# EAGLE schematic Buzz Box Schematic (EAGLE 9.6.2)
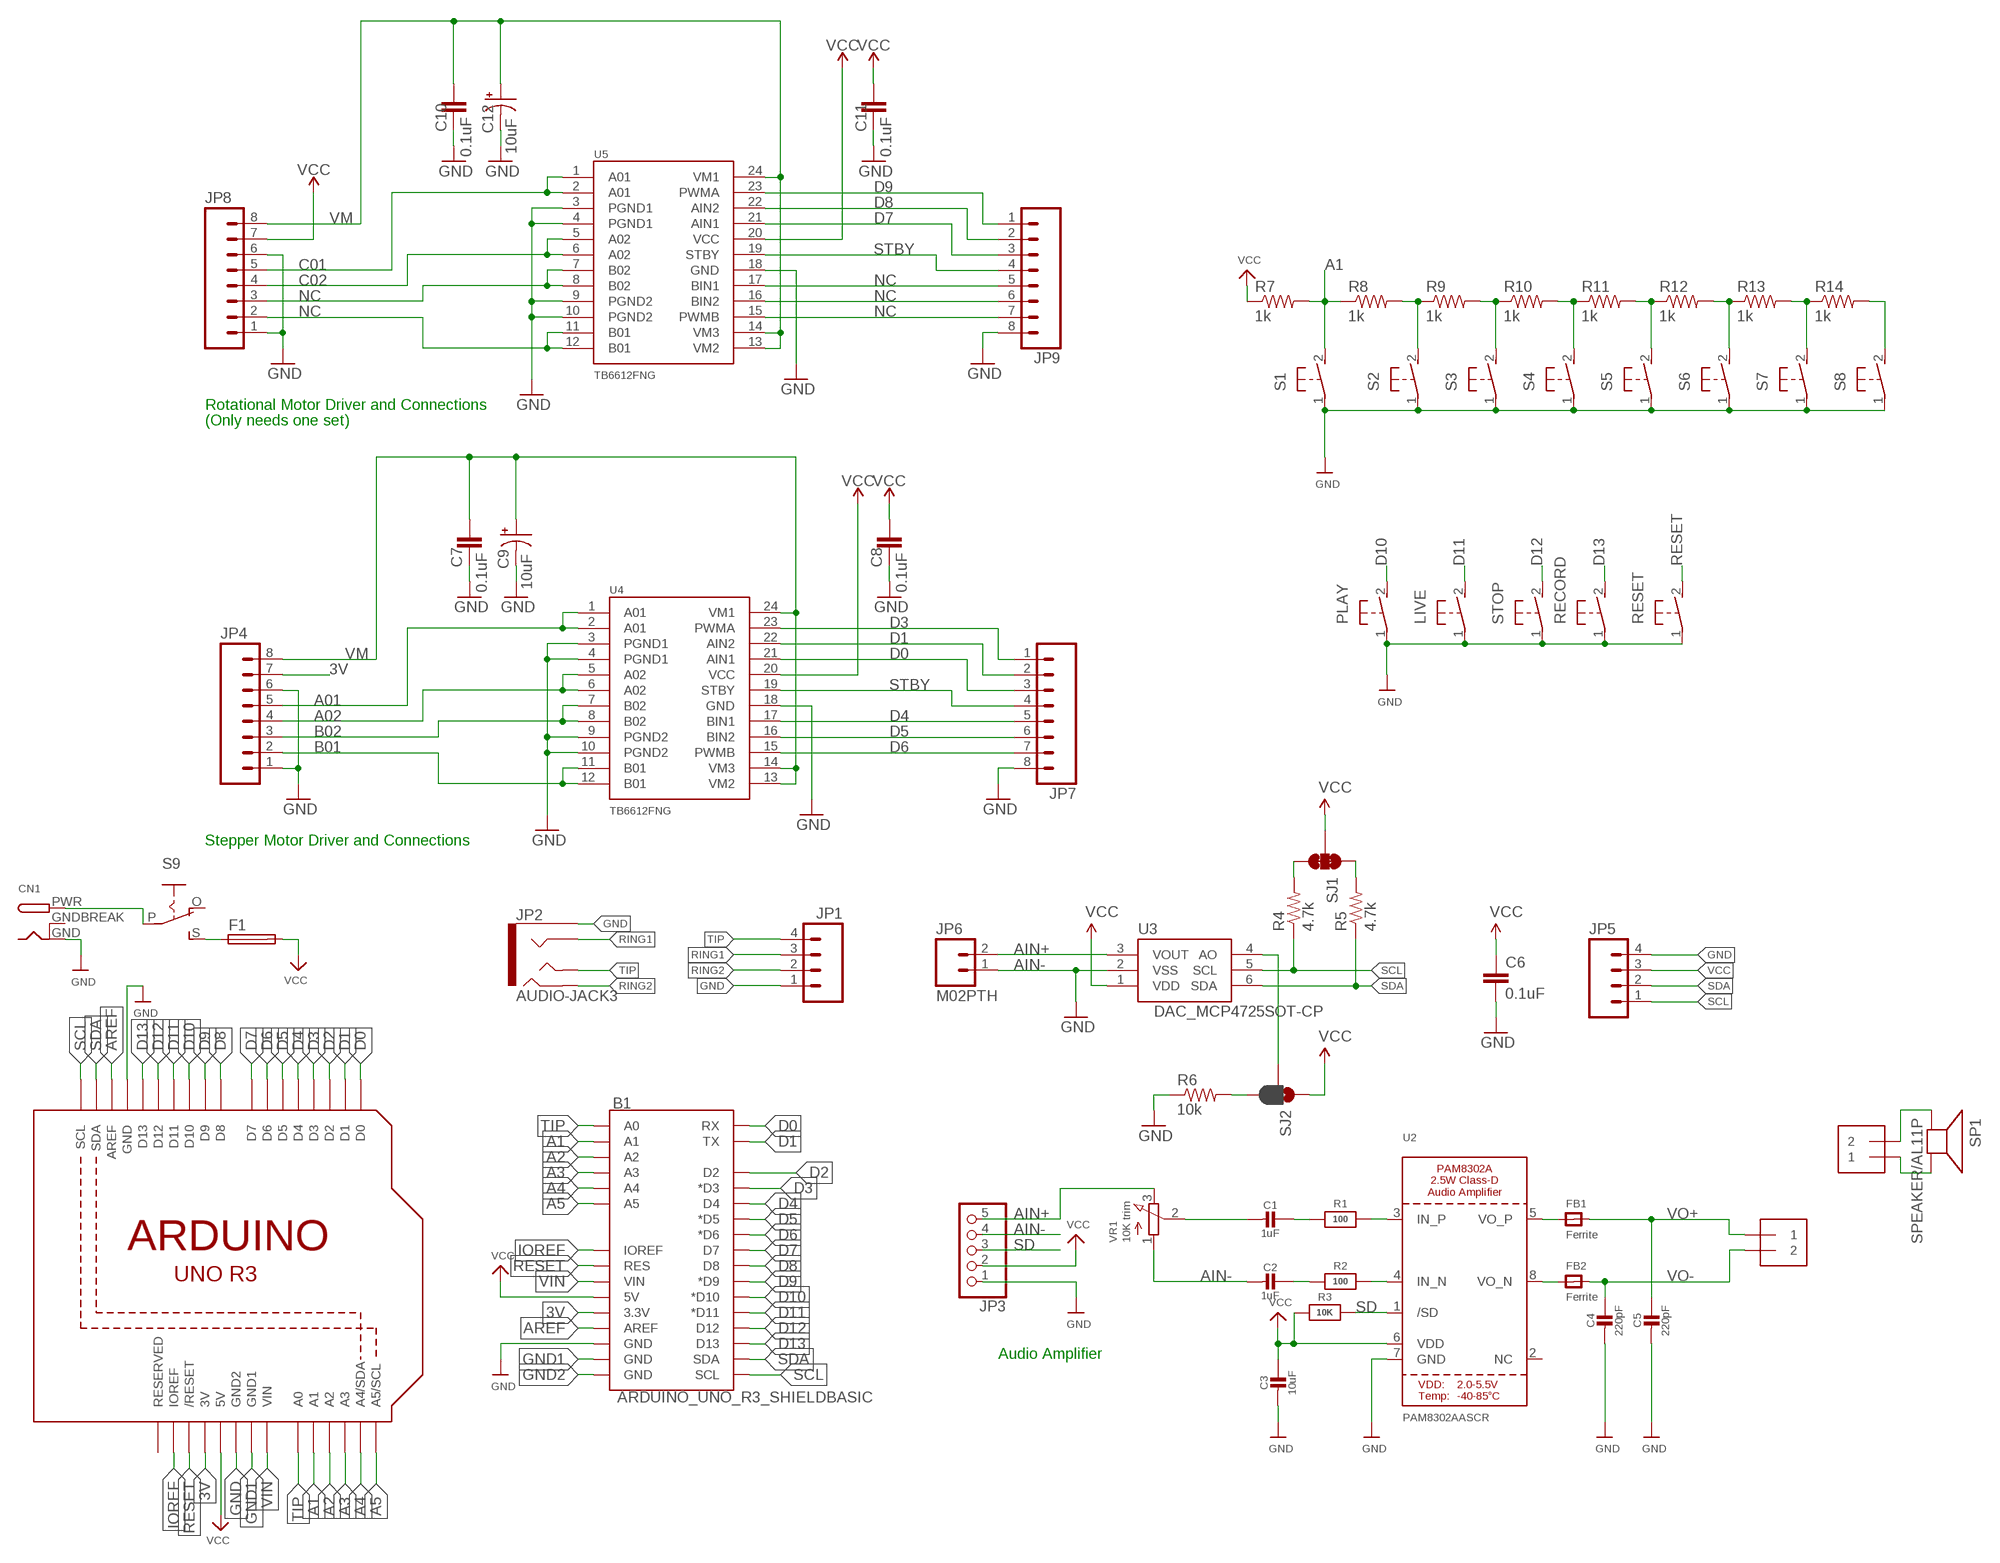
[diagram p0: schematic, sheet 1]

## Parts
B1  ARDUINO_UNO_R3_SHIELDBASIC  [UNO_R3_SHIELD]
C1  1uF  CAP_CERAMIC0805-NOOUTLINE  [0805-NO]
C2  1uF  CAP_CERAMIC0805-NOOUTLINE  [0805-NO]
C3  10uF  CAP_CERAMIC0805-NOOUTLINE  [0805-NO]
C4  220pF  CAP_CERAMIC0805-NOOUTLINE  [0805-NO]
C5  220pF  CAP_CERAMIC0805-NOOUTLINE  [0805-NO]
C6  0.1uF  CAP0603-CAP  [0603-CAP]
C7  0.1uF  0.1UF-0402-16V-10%  [0402]
C8  0.1uF  0.1UF-0402-16V-10%  [0402]
C9  10uF  10UF-POLAR-EIA3528-20V-10%(TANT)  [EIA3528]
C10  0.1uF  0.1UF-0402-16V-10%  [0402]
C11  0.1uF  0.1UF-0402-16V-10%  [0402]
C12  10uF  10UF-POLAR-EIA3528-20V-10%(TANT)  [EIA3528]
CN1  DCBARRELPTH  [DCJACK_2MM_PTH]
F1  19560  [19560]
FB1  Ferrite  FERRITE_0805  [_0805]
FB2  Ferrite  FERRITE_0805  [_0805]
JP1  M04PTH  [1X04]
JP2  AUDIO-JACK3  [AUDIO-JACK-TRRS-SMD]
JP3  HEADER-1X570MIL  [1X05_ROUND_70]
JP4  M0875_PERCENT_REDUCED  [1X08_OFFSET_REDUCED]
JP5  M04PTH  [1X04]
JP6  M02PTH  [1X02]
JP7  M0875_PERCENT_REDUCED  [1X08_OFFSET_REDUCED]
JP8  M0875_PERCENT_REDUCED  [1X08_OFFSET_REDUCED]
JP9  M0875_PERCENT_REDUCED  [1X08_OFFSET_REDUCED]
LIVE  31-XX  [B3F-31XX]
PLAY  31-XX  [B3F-31XX]
R1  100  RESISTOR0805_NOOUTLINE  [0805-NO]
R2  100  RESISTOR0805_NOOUTLINE  [0805-NO]
R3  10K  RESISTOR0805_NOOUTLINE  [0805-NO]
R4  4.7k  RESISTOR0603-RES  [0603-RES]
R5  4.7k  RESISTOR0603-RES  [0603-RES]
R6  10k  RESISTOR0603-RES  [0603-RES]
R7  1k  R-US_0817/22  [P0817/22]
R8  1k  R-US_0817/22  [P0817/22]
R9  1k  R-US_0817/22  [P0817/22]
R10  1k  R-US_0817/22  [P0817/22]
R11  1k  R-US_0817/22  [P0817/22]
R12  1k  R-US_0817/22  [P0817/22]
R13  1k  R-US_0817/22  [P0817/22]
R14  1k  R-US_0817/22  [P0817/22]
RECORD  31-XX  [B3F-31XX]
RESET  31-XX  [B3F-31XX]
S1  31-XX  [B3F-31XX]
S2  31-XX  [B3F-31XX]
S3  31-XX  [B3F-31XX]
S4  31-XX  [B3F-31XX]
S5  31-XX  [B3F-31XX]
S6  31-XX  [B3F-31XX]
S7  31-XX  [B3F-31XX]
S8  31-XX  [B3F-31XX]
S9  EG1218S  [EG1218]
SJ1  JUMPER-PAD-3-NC_BY_TRACE  [PAD-JUMPER-3-3OF3_NC_BY_TRACE_YES_SILK_FULL_BOX]
SJ2  JUMPER-PAD-3-2OF3_NC_BY_PASTE  [PAD-JUMPER-3-2OF3_NC_BY_PASTE_YES_SILK_FULL_BOX]
SP1  SPEAKER/AL11P  [AL11P]
STOP  31-XX  [B3F-31XX]
U1  ARDUINOR3-BPLACE  [ARDUINOR3-BPLACE]
U2  PAM8302AASCR  AUDIOAMP_PAM8302A  [MSOP8_0.65MM]
U3  DAC_MCP4725SOT-CP  [SOT23-6-MCP4725]
U4  TB6612FNG  [SSOP24]
U5  TB6612FNG  [SSOP24]
VR1  10K trim  TRIMPOT3303W/X  [TRIMPOT_BOURNS_3303W]
X1  TERMBLOCK_1X2  [TERMBLOCK_1X2-3.5MM]
X2  TERMBLOCK_1X2  [TERMBLOCK_1X2-3.5MM]

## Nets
3V: B1.3.3V JP4.7 U1.3V
A1: B1.A1 R7.2 R8.1 S1.2(S) U1.A1
A01: JP4.5 U4.1(A01) U4.2(A01)
A2: B1.A2 U1.A2
A02: JP4.4 U4.5(A02) U4.6(A02)
A3: B1.A3 U1.A3
A4: B1.A4 U1.A4(A4/SDA)
A5: B1.A5 U1.A5(A5/SCL)
AIN+: JP3.5 JP6.2 U3.3(VOUT) VR1.3(E)
AIN-: C2.2 JP3.4 JP6.1 U3.2(VSS) VR1.1(A) ; supply symbol labelled GND
AREF: B1.AREF U1.AREF
B01: JP4.2 U4.11(B01) U4.12(B01)
B02: JP4.3 U4.7(B02) U4.8(B02)
C01: JP8.5 U5.1(A01) U5.2(A01)
C02: JP8.4 U5.5(A02) U5.6(A02)
D0: B1.RX JP7.3 U1.D0 U4.21(AIN1)
D1: B1.TX JP7.2 U1.D1 U4.22(AIN2)
D2: B1.D2 U1.D2
D3: B1.D3(*D3) JP7.1 U1.D3 U4.23(PWMA)
D4: B1.D4 JP7.5 U1.D4 U4.17(BIN1)
D5: B1.D5(*D5) JP7.6 U1.D5 U4.16(BIN2)
D6: B1.D6(*D6) JP7.7 U1.D6 U4.15(PWMB)
D7: B1.D7 JP9.3 U1.D7 U5.21(AIN1)
D8: B1.D8 JP9.2 U1.D8 U5.22(AIN2)
D9: B1.D9(*D9) JP9.1 U1.D9 U5.23(PWMA)
D10: B1.D10(*D10) PLAY.2(S) U1.D10
D11: B1.D11(*D11) LIVE.2(S) U1.D11
D12: B1.D12 STOP.2(S) U1.D12
D13: B1.D13 RECORD.2(S) U1.D13
GND: B1.GND@2(GND) C3.2 C4.2 C5.2 C6.2 C7.2 C8.2 C9.C(-) C10.2 C11.2 C12.C(-) CN1.GND JP1.1 JP2.EARTH JP3.1 JP4.1 JP4.6 JP5.4 JP7.8 JP8.1 JP8.6 JP9.8 LIVE.1(P) PLAY.1(P) R6.1 RECORD.1(P) RESET.1(P) S1.1(P) S2.1(P) S3.1(P) S4.1(P) S5.1(P) S6.1(P) S7.1(P) S8.1(P) STOP.1(P) U1.GND U1.GND2 U2.7(GND) U4.3(PGND1) U4.4(PGND1) U4.9(PGND2) U4.10(PGND2) U4.18(GND) U5.3(PGND1) U5.4(PGND1) U5.9(PGND2) U5.10(PGND2) U5.18(GND)
GND1: B1.GND@1(GND) U1.GND1
GND2: B1.GND@0(GND)
IOREF: B1.IOREF U1.IOREF
N$1: R2.2 U2.4(IN_N)
N$2: R1.2 U2.3(IN_P)
N$3: C1.1 R1.1
N$4: C2.1 R2.1
N$5: FB2.1 U2.8(VO_N)
N$6: FB1.1 U2.5(VO_P)
N$7: C1.2 VR1.2(S)
N$8: R5.2 SJ1.1
N$9: R4.2 SJ1.3
N$10: SJ2.2 U3.4(AO)
N$11: R6.2 SJ2.3
N$12: SP1.+ X2.2
N$13: SP1.- X2.1
N$14: CN1.PWR S9.P
N$15: R8.2 R9.1 S2.2(S)
N$16: R9.2 R10.1 S3.2(S)
N$17: R10.2 R11.1 S4.2(S)
N$18: R11.2 R12.1 S5.2(S)
N$19: R12.2 R13.1 S6.2(S)
N$20: R13.2 R14.1 S7.2(S)
N$21: R14.2 S8.2(S)
N$22: F1.1 S9.S
NC: JP8.2 JP8.3 JP9.5 JP9.6 JP9.7 U5.7(B02) U5.8(B02) U5.11(B01) U5.12(B01) U5.15(PWMB) U5.16(BIN2) U5.17(BIN1)
RESET: B1.RES RESET.2(S) U1.RESET(/RESET)
RING1: JP1.3 JP2.RING1
RING2: JP1.2 JP2.RING2
SCL: B1.SCL JP5.1 R4.1 U1.SCL U3.5(SCL)
SD: JP3.3 R3.2 U2.1(/SD)
SDA: B1.SDA JP5.2 R5.1 U1.SDA U3.6(SDA)
STBY: JP7.4 JP9.4 U4.19(STBY) U5.19(STBY)
TIP: B1.A0 JP1.4 JP2.TIP U1.A0
VCC: B1.5V C3.1 C6.1 C8.1 C11.1 F1.2 JP3.2 JP5.3 JP8.7 R3.1 R7.1 SJ1.2 SJ2.1 U1.5V U2.6(VDD) U3.1(VDD) U4.20(VCC) U5.20(VCC)
VIN: B1.VIN U1.VIN
VM: C7.1 C9.A(+) C10.1 C12.A(+) JP4.8 JP8.8 U4.13(VM2) U4.14(VM3) U4.24(VM1) U5.13(VM2) U5.14(VM3) U5.24(VM1)
VO+: C5.1 FB1.2 X1.1
VO-: C4.1 FB2.2 X1.2
Unconnected: S9.O U1.RESERVED U2.2(NC)

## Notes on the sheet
- Rotational Motor Driver and Connections
- (Only needs one set)
- Stepper Motor Driver and Connections
- Audio Amplifier

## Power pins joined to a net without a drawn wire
GNDBREAK: CN1.GNDBREAK

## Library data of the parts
B1 = SparkFun-Boards:ARDUINO_UNO_R3_SHIELD: Arduino R3 Shield Footprint Shield form compatible with the Arduino Uno R3. SparkFun Products: MG2639 Cellular Shield MIDI Shield R3 Stackable Headers Kit
C1-C5 = microbuilder:CAP_CERAMIC: Ceramic Capacitors
C6 = SparkFun:CAP: Capacitor
C7 C8 C10 C11 = SparkFun-Capacitors:0.1UF: 0.1µF ceramic capacitors; PROD_ID: CAP-12416
C9 C12 = SparkFun-Capacitors:10UF-POLAR: 10.0µF polarized capacitors; PROD_ID: CAP-08063
CN1 = adafruit:DCBARREL: 2.0mm DC Barrel Jack DCJACK_2MM_PTH - Through Hole Jack (4UConnector: 05537)
F1 = fuse:19560: FUSE HOLDER; MPN: 56000001009; OC_FARNELL: 1185363; OC_NEWARK: 15P8392
FB1 FB2 = microbuilder:FERRITE: Ferrite Bead
JP1 JP5 = SparkFun-Connectors:M04: Header 4 Standard 4-pin 0.1" header. Use with straight break away headers (SKU : PRT-00116), right angle break away headers (PRT-00553), swiss pins (PRT-00743), machine pins (PRT-00117), and female headers (PRT-00115). Molex polarized connector foot print use with SKU : PRT-08231 with associated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
JP2 = SparkFun-Connectors:AUDIO-JACK3: Audio jack - 3.5mm TRRS variety - two rings.
JP3 = microbuilder:HEADER-1X5: PIN HEADER
JP4 JP7-JP9 = Testing:M08: Header 8 Standard 8-pin 0.1" header. Use with straight break away headers (SKU : PRT-00116), right angle break away headers (PRT-00553), swiss pins (PRT-00743), machine pins (PRT-00117), and female headers (PRT-00115).
JP6 = SparkFun-Connectors:M02: Standard 2-pin 0.1" header. Use with
LIVE PLAY RECORD RESET STOP = adafruit:31-XX: OMRON SWITCH
R1-R3 = microbuilder:RESISTOR: Resistors
R4-R6 = SparkFun:RESISTOR: Resistor
R7-R14 = rcl:R-US_: RESISTOR, American symbol; SPICEPREFIX: R
S1-S8 = adafruit:31-XX: OMRON SWITCH; SPICEPREFIX: B
S9 = adafruit:EG1218: SLIDING SWITCH 0.1" spacing through hole, vertical SPDT slide switch http://www.ladyada.net/library/pcb/eaglelibrary.html
SJ1 = SparkFun-Passives:JUMPER-PAD-3-NC_BY_TRACE
SJ2 = SparkFun-Passives:JUMPER-PAD-3-2OF3_NC_BY_PASTE
SP1 = adafruit:SPEAKER: SPEAKER
U1 = adafruit:ARDUINOR3: This is a new object for the new Arduino R3 - with extra pins that you may want to use (such as IOref, and duplicated A4/A5
U2 = microbuilder:AUDIOAMP_PAM8302A: PAM8302A - 2.5W Class-D Mono Audio Amplifier MSOP8 = PAM8302AASCR
U3 = SparkFun-AnalogIC:DAC_MCP4725: Microchip 12-bit I2C DAC, SOT23-6
U4 U5 = SparkFun-IC-Special-Function:TB6612FNG: Toshiba 1A dual motor driver IC-09363; PROD_ID: IC-09363
VR1 = microbuilder:TRIMPOT: 3-Pin SMT Trimpots Bourns TC33 (X-2) Series 1K - Digikey: TC33X-102ECT-ND 10K - Digikey: TC33X-2-103E 100K - Digikey: TC33X-104ECT-ND Bourns 3303 (W) Series 3mm 10K Single Turn - Digikey: 3303W-103ETR-ND 3mm 100K Single Turn - Digikey: 3303X-104ETR-ND
X1 X2 = microbuilder:TERMBLOCK_1X2: 3.5mm Terminal block

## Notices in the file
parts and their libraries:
SparkFun-Boards: Licensing: Creative Commons ShareAlike 4.0 International - https://creativecommons.org/licenses/by-sa/4.0
SparkFun-Connectors: Licensing: CC v3.0 Share-Alike You are welcome to use this library for commercial purposes.
